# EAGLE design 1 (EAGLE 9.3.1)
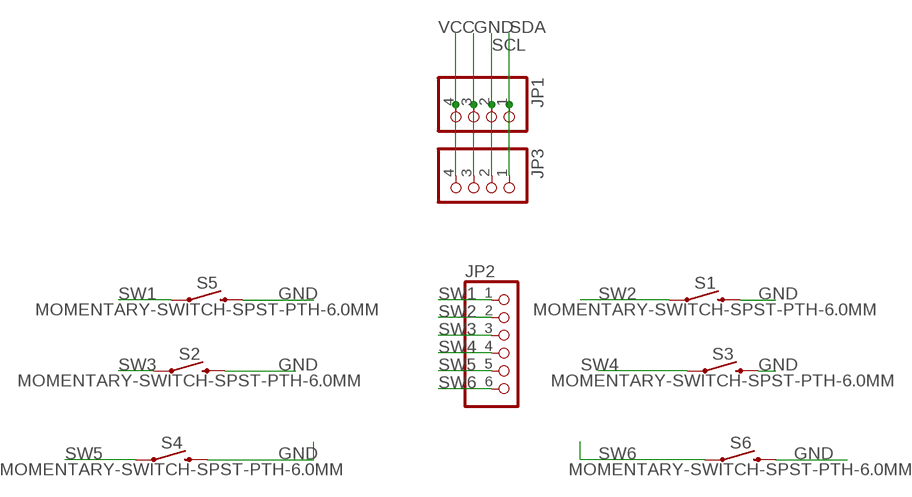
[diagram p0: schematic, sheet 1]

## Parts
JP1  PINHD-1X4  [1X04]
JP2  PINHD-1X6  [1X06]
JP3  PINHD-1X4  [1X04]
S1  MOMENTARY-SWITCH-SPST-PTH-6.0MM  [TACTILE_SWITCH_PTH_6.0MM]
S2  MOMENTARY-SWITCH-SPST-PTH-6.0MM  [TACTILE_SWITCH_PTH_6.0MM]
S3  MOMENTARY-SWITCH-SPST-PTH-6.0MM  [TACTILE_SWITCH_PTH_6.0MM]
S4  MOMENTARY-SWITCH-SPST-PTH-6.0MM  [TACTILE_SWITCH_PTH_6.0MM]
S5  MOMENTARY-SWITCH-SPST-PTH-6.0MM  [TACTILE_SWITCH_PTH_6.0MM]
S6  MOMENTARY-SWITCH-SPST-PTH-6.0MM  [TACTILE_SWITCH_PTH_6.0MM]

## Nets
GND: JP1.3 JP3.3 S1.3 S2.3 S3.3 S4.3 S5.3 S6.3
SCL: JP1.2 JP3.2
SDA: JP1.1 JP3.1
SW1: JP2.1 S5.1
SW2: JP2.2 S1.1
SW3: JP2.3 S2.1
SW4: JP2.4 S3.1
SW5: JP2.5 S4.1
SW6: JP2.6 S6.1
VCC: JP1.4 JP3.4

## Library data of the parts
JP1 JP3 = pinhead:PINHD-1X4: PIN HEADER
JP2 = pinhead:PINHD-1X6: PIN HEADER
S1-S6 = SparkFun-Switches:MOMENTARY-SWITCH-SPST: Momentary Switch (Pushbutton) - SPST; PROD_ID: SWCH-08441; SF_SKU: COM-00097

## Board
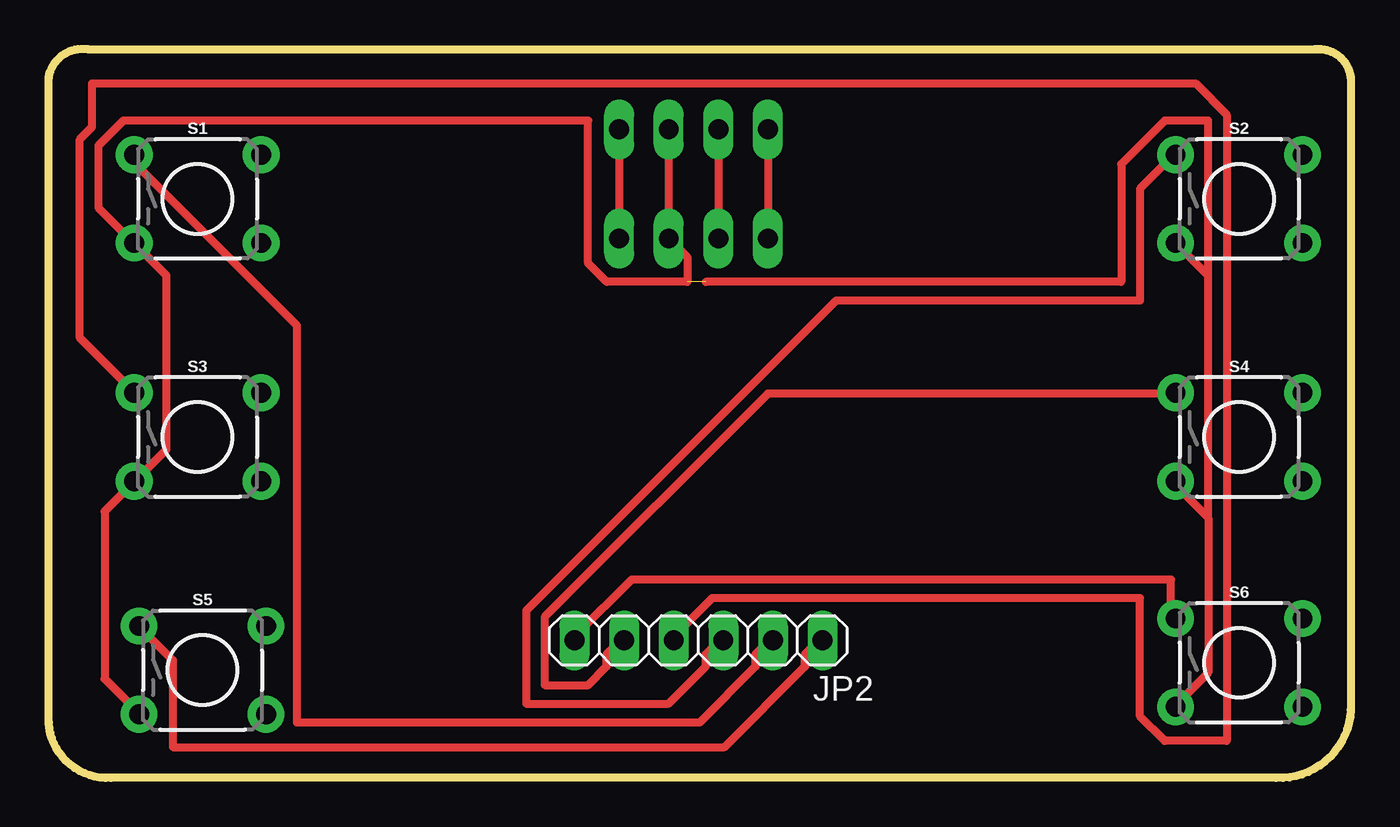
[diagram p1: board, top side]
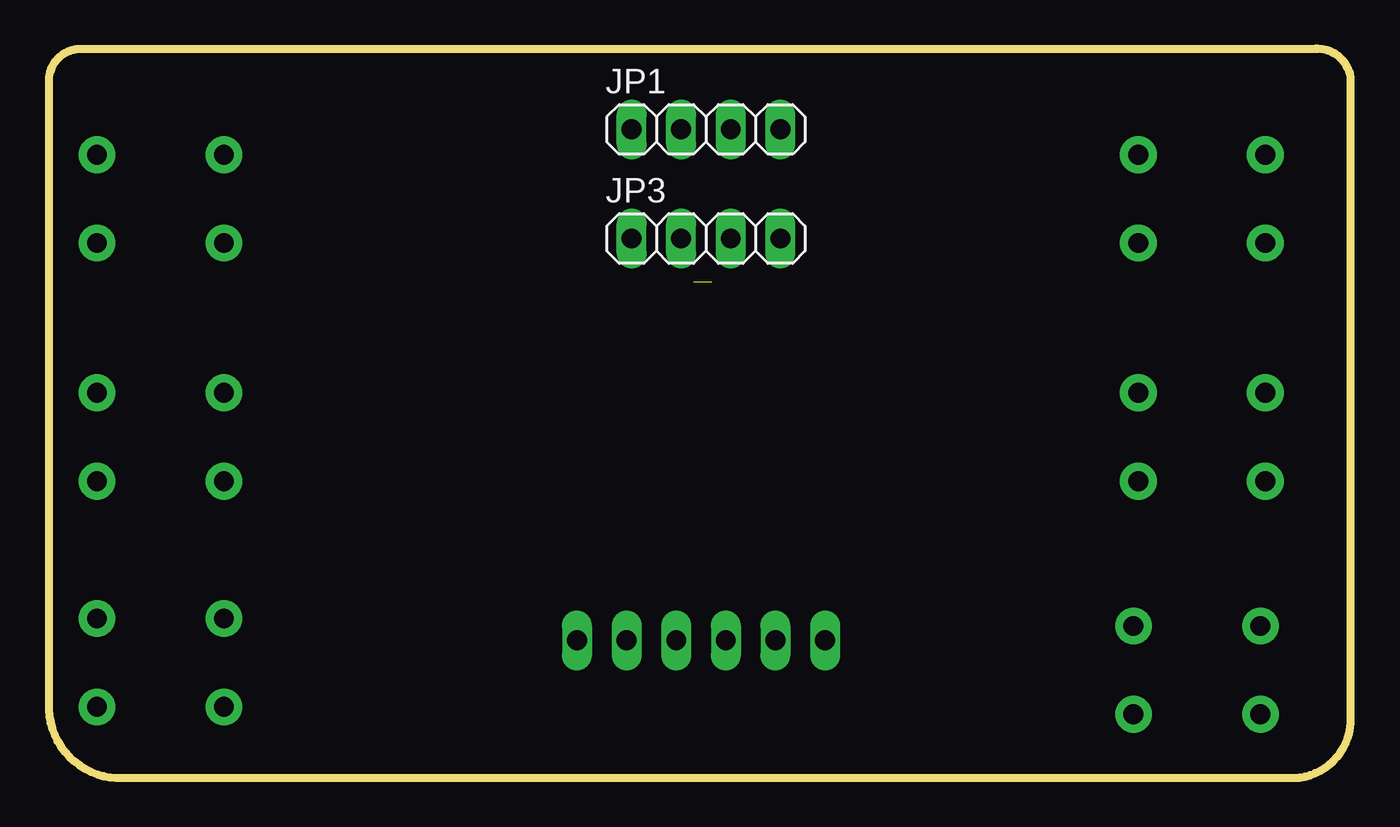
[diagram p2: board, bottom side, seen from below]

Size 66.67 x 37.33 mm. Coordinates in mm from the lower left corner, seen from the top.
Outline: 62.87,0 3.17,0 arc-90 0,2.85 0,35.87 arc-90 1.98,37.31 64.85,37.31 arc-90 66.67,35.87 66.67,3.49 arc-90 62.87,0
Copper layers (1*16): Top 0.035mm / dielectric 1.5mm / Bottom 0.035mm
Design rules "default *": minimum track width 16mil, minimum drill 0.35mm, track to track 16mil, track to pad 16mil, pad to pad 16mil, via to via 16mil, smd to smd 16mil, copper to edge 40mil, drill to drill 6mil, minimum pad ring 10mil, minimum via ring 8mil, stop-mask expansion 4mil, vias tented up to drill 0mil, thermal gap 10mil

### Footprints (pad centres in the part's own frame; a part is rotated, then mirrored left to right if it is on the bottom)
1X04 = drill 1.016 long: 1 -3.81,0; 2 -1.27,0; 3 1.27,0; 4 3.81,0
1X06 = drill 1.016 long: 1 -6.35,0; 2 -3.81,0; 3 -1.27,0; 4 1.27,0; 5 3.81,0; 6 6.35,0
TACTILE_SWITCH_PTH_6.0MM = drill 1.016 pad 1.88: 1 -3.251,2.261; 2 3.251,2.261; 3 -3.251,-2.261; 4 3.251,-2.261

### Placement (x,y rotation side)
JP1  33.02,33.2 0 bottom
JP2  33.27,7.04 180 top
JP3  33.02,27.62 0 bottom
S1  7.62,29.65 0 top
S2  60.96,29.65 0 top
S3  7.62,17.46 0 top
S4  60.96,17.46 0 top
S5  7.87,5.52 0 top
S6  60.96,5.9 0 top

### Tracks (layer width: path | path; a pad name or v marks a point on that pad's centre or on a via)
GND  (1 unrouted)
  Top 0.406: S5.3 4.44,3.49 2.86,5.07 2.86,13.65 4.13,14.92 S3.3 4.44,15.23 6.03,16.82 6.03,25.71 4.44,27.3 S1.3 4.13,27.62 2.54,29.2 2.54,32.38 3.81,33.65 27.62,33.65 27.62,26.35 28.57,25.39 32.7,25.39 32.7,26.66 JP3.3 JP1.3 | 59.37,13.33 59.37,5.39 57.79,3.8 S6.3 | 59.37,13.33 57.79,14.92 S4.3 | 59.37,25.71 57.79,27.3 S2.3 | 59.37,13.33 59.37,25.71 | 33.66,25.39 54.93,25.39 54.93,31.43 57.15,33.65 59.37,33.65 59.37,25.71
SCL
  Top 0.406: JP1.2 JP3.2
SDA
  Top 0.406: JP1.1 JP3.1
SW1
  Top 0.406: JP2.1 39.37,6.98 38.73,6.34 38.73,5.71 34.61,1.58 6.35,1.58 6.35,6.03 4.76,7.61 S5.1
SW2
  Top 0.406: JP2.2 36.83,6.98 36.2,6.34 36.2,5.71 33.34,2.85 12.7,2.85 12.7,23.17 4.44,31.43 4.44,31.74 S1.1
SW3
  Top 0.406: JP2.3 34.29,6.98 33.66,6.34 33.66,5.71 31.75,3.8 24.45,3.8 24.45,8.57 40.32,24.44 55.88,24.44 55.88,30.16 57.47,31.74 S2.1
SW4
  Top 0.406: JP2.4 32.07,7.3 33.97,9.2 55.88,9.2 55.88,3.17 57.15,1.9 60.32,1.9 60.32,33.97 58.74,35.55 2.22,35.55 2.22,33.33 1.59,32.7 1.59,22.54 4.13,20 S3.1
SW5
  Top 0.406: JP2.5 29.21,6.98 28.57,6.34 28.57,5.71 27.62,4.76 25.4,4.76 25.4,8.25 36.83,19.68 57.47,19.68 S4.1
SW6
  Top 0.406: JP2.6 26.99,7.3 29.85,10.15 57.47,10.15 57.47,8.25 S6.1
VCC
  Top 0.406: JP1.4 JP3.4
